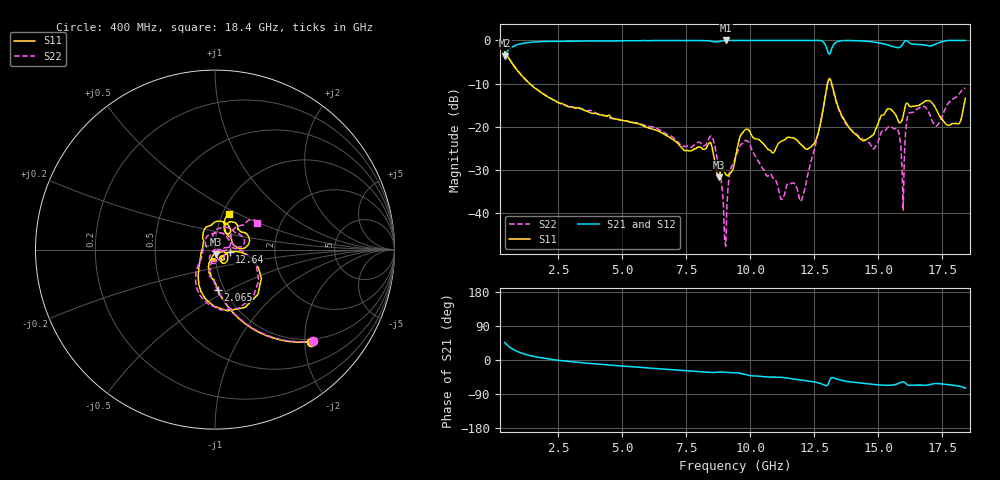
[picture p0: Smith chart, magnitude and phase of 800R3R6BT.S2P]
!  American Technical Ceramics  Date:  10/25/10
!  One Norden Lane
!  Huntington Station,  NY.  11746-2102
!  Tel:  (631) 622-4700  Fax:  (631) 622-4748
!  Part Number  800R3R6BT  Mounting Orientation: Vertical
!  Description: Ultra Low ESR Microwave Capacitor
!  Application: Coupling, Bypass, Tuning, DC Block, Filters, Matching
# GHZ S DB R 50
! Freq  |S11|  S11 Ph  |S21|  S21 Ph  |S12|  S12 Ph  |S22|  S22 Ph
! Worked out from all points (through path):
!   401 points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, 400 MHz to 18.4 GHz, reference 50 ohm
!   highest |S21| = -0.01 dB at 9.04 GHz (marker M1); lowest = -3.6 dB at 400 MHz (marker M2)
!   group delay of S21, straight-line fit = 13.8 ps
!   lowest |S11| = -31.8 dB at 8.77 GHz (marker M3), VSWR 1.05, Z = 50.3 - j2.57 ohm
!   |S11| at or under -10 dB: 1.371 GHz to 13.01 GHz (11.64 GHz wide, 162 % of centre); 13.18 GHz to end of sweep
!   |S22| runs from -47.8 to -2.5 dB; largest |S21 - S12| = 0.005
!   S11 on the Smith chart (normalised r, x): 400 MHz: 0.94, -2.14; 2.065 GHz: 0.93, -0.44; 12.64 GHz: 1.18, -0.03; 18.4 GHz: 1.07, +0.45
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0.4  -2.61 -43.8  -3.56 46.1  -3.58 46.1  -2.55 -43.1
2.065  -13.01 -86.2  -0.23 3.2  -0.26 3.3  -13.03 -87.0
3.415  -15.91 -96.6  -0.14 -7.1  -0.15 -7.0  -15.97 -96.7
6.43  -21.08 -112.8  -0.04 -23.0  -0.04 -22.9  -20.68 -105.5
8.455  -23.81 -101.6  -0.17 -33.2  -0.15 -33.1  -22.16 -95.3
8.77  -31.77 -81.1  -0.26 -31.7  -0.24 -31.6  -29.75 -130.6
9.04  -31.14 -67.7  -0.01 -32.3  -0.01 -32.1  -47.75 49.4
9.4  -27.72 -16.5  -0.01 -33.5  -0.01 -33.3  -27.52 -14.3
9.85  -20.61 -47.2  -0.01 -38.9  -0.01 -38.8  -23.28 -51.4
11.2  -23.46 -42.7  -0.01 -45.8  -0.01 -45.8  -36.93 -62.8
11.965  -24.11 -54.4  -0.01 -53.0  -0.01 -53.0  -37.36 -31.0
12.415  -24.38 -27.8  -0.01 -56.7  -0.01 -56.8  -27.10 10.1
12.64  -21.70 -10.2  -0.01 -60.0  -0.01 -60.0  -21.87 8.2
13.09  -8.81 -62.7  -3.24 -55.1  -3.23 -55.2  -9.04 -68.2
14.35  -23.06 175.0  -0.12 -61.2  -0.09 -61.3  -22.69 -163.8
15.43  -15.87 73.4  -1.18 -67.0  -1.16 -67.2  -20.00 62.7
15.745  -18.17 48.3  -1.68 -63.0  -1.65 -63.1  -20.46 22.0
15.925  -18.58 63.2  -1.11 -57.6  -1.10 -57.9  -29.82 -11.3
16.24  -15.37 42.1  -0.69 -66.9  -0.66 -67.0  -16.76 50.3
17.275  -16.20 1.9  -0.76 -62.1  -0.74 -62.3  -19.87 25.8
18.085  -19.38 42.2  -0.01 -68.0  -0.01 -68.2  -12.92 40.8
18.4  -13.38 69.5  -0.01 -74.3  -0.01 -74.5  -11.14 32.1
